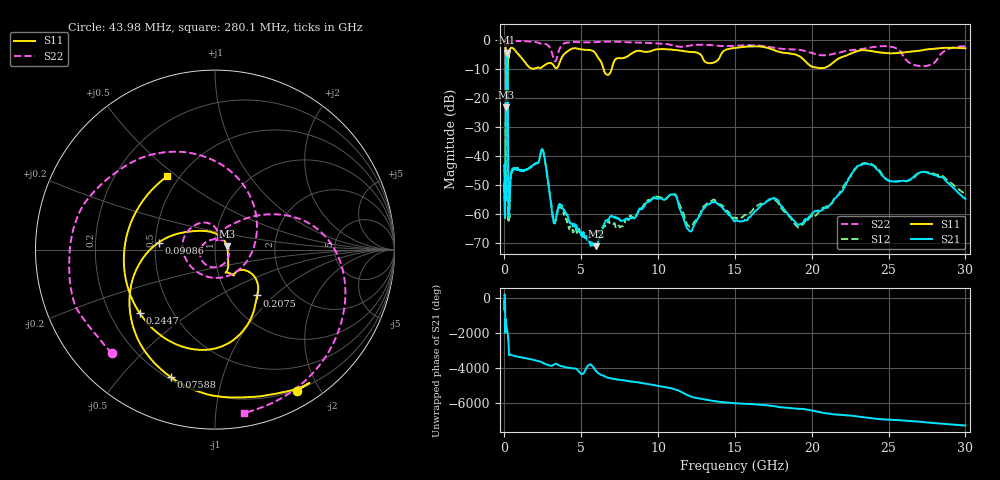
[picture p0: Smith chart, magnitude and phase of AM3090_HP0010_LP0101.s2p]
! Date/Time: Thu, Feb 28, 2019 1:55 PM
! Network Analyzer: Agilent Technologies E8364B Rev: A.07.50.67
! Sweep from 0.010 to 30.000 GHz, 1601 Points, Sweep Type: LOG
! Power Supply: 5.022 V, 0.002 A
# Hz S DB R 50
!freq MagS11 AngS11 MagS21 AngS21 MagS12 AngS12 MagS22 AngS22
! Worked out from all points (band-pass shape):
!   1601 points, 10 MHz to 30 GHz, reference 50 ohm
!   highest |S21| = -4.37 dB at 144 MHz (marker M1); lowest = -71.1 dB at 5.989 GHz (marker M2)
!   |S21| within 3 dB of the highest: 101.1 MHz to 201.4 MHz (100.3 MHz wide, 66.3 % of centre)
!   lowest |S11| = -23.2 dB at 99.43 MHz (marker M3), VSWR 1.15, Z = 57 + j2.34 ohm
!   |S11| at or under -10 dB: 90.88 MHz to 202.7 MHz (111.8 MHz wide, 76.2 % of centre); 6.451 GHz to 6.979 GHz (527.5 MHz wide, 7.86 % of centre)
!   |S22| runs from -26.4 to -0.2 dB; largest |S21 - S12| = 0.012
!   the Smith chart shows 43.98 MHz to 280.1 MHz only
!   S11 on the Smith chart (normalised r, x): 43.98 MHz: 0.18, -1.72; 75.88 MHz: 0.21, -0.69; 90.86 MHz: 0.52, +0.05; 207.5 MHz: 1.35, -0.79; 244.7 MHz: 0.33, -0.33; 280.1 MHz: 0.43, +0.46
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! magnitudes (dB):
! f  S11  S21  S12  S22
! 10 MHz  -0.2  -43.4  -45.6  -0.5
! 38.04 MHz  -0.5  -58.6  -60.5  -1.4
! 43.98 MHz  -0.8  -57.7  -60.0  -1.8
! 75.88 MHz  -2.5  -47.9  -48.9  -4.6
! 90.86 MHz  -10.0  -15.9  -15.8  -15.8
! 99.43 MHz  -23.2  -8.0  -7.9  -14.6
! 144 MHz  -15.5  -4.4  -4.3  -22.6
! 144.7 MHz  -15.5  -4.4  -4.3  -22.4
! 207.5 MHz  -9.2  -8.9  -8.9  -15.5
! 244.7 MHz  -5.2  -52.9  -55.3  -1.6
! 280.1 MHz  -6.2  -61.0  -62.2  -0.7
! 550.5 MHz  -2.9  -45.1  -44.7  -0.2
! 2.084 GHz  -9.7  -42.4  -42.5  -0.8
! 2.52 GHz  -9.0  -38.3  -38.3  -1.3
! 3.236 GHz  -9.0  -63.2  -62.1  -7.1
! 5.989 GHz  -5.2  -71.1  -65.8  -0.7
! 7.926 GHz  -5.9  -61.6  -61.8  -0.7
! 10.81 GHz  -3.3  -53.3  -53.3  -1.7
! 12.07 GHz  -4.1  -66.0  -64.5  -1.9
! 19.51 GHz  -6.9  -62.1  -63.1  -3.7
! 23.48 GHz  -3.5  -42.6  -42.4  -2.9
! 30 GHz  -2.9  -54.8  -53.4  -2.2
